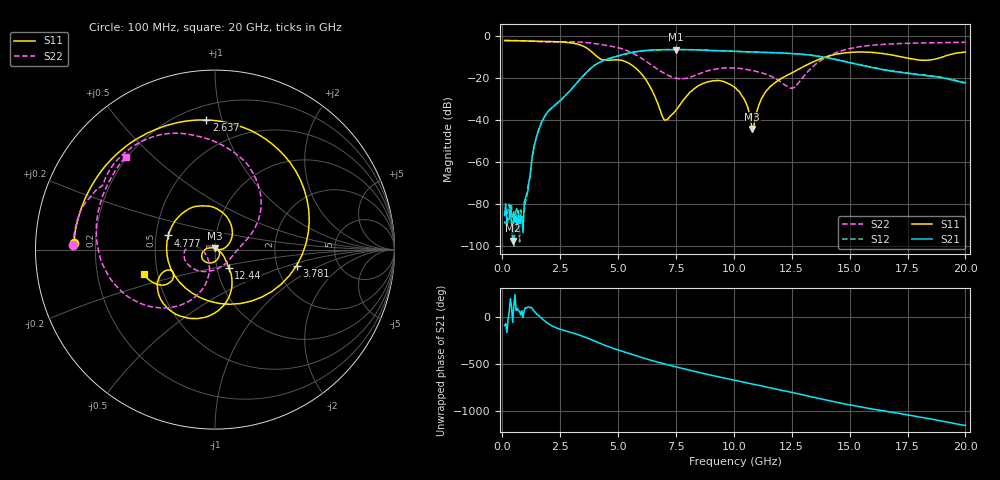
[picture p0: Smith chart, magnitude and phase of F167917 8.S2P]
!  2-Port S-parameters saved by WinCal
! VAR MeasName=S-Parameters (CALIBRATED_DATA) read from VNA (N5242A)
! VAR MeasDate=2016-11-22 9:00:03
! VAR NAME=F167917 8
! VAR FILENAME=F167917 8.S2P
! VAR DATE=2016-11-22 9:00:03
! VAR PHYS_PORTS=1,2
# Hz S DB R 50
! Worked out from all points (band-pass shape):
!   401 points, 100 MHz to 20 GHz, reference 50 ohm
!   highest |S21| = -6.37 dB at 7.513 GHz (marker M1); lowest = -97.2 dB at 448.2 MHz (marker M2)
!   |S21| within 3 dB of the highest: 5.017 GHz to 13.54 GHz (8.526 GHz wide, 91.9 % of centre)
!   lowest |S11| = -44.2 dB at 10.8 GHz (marker M3), VSWR 1.01, Z = 50.1 + j0.616 ohm
!   |S11| at or under -10 dB: 4.127 GHz to 13.93 GHz (9.808 GHz wide, 109 % of centre); 17.32 GHz to 18.97 GHz (1.658 GHz wide, 9.14 % of centre)
!   |S22| runs from -24.7 to -2.0 dB; largest |S21 - S12| = 0.0043
!   S11 on the Smith chart (normalised r, x): 100 MHz: 0.12, +0.02; 2.637 GHz: 0.29, +0.89; 3.781 GHz: 2.57, -0.59; 4.777 GHz: 0.58, +0.10; 12.44 GHz: 1.14, -0.24; 20 GHz: 0.42, -0.14
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1e8  -2.09 177.3  -85.30 -87.7  -87.89 150.7  -2.03 178.3
4.4825e8  -2.13 168.0  -97.22 -53.9  -89.70 -97.5  -2.06 172.4
9.4575e8  -2.21 154.7  -79.15 73.5  -84.02 95.0  -2.18 163.9
1.5925e9  -2.34 135.6  -43.93 12.3  -43.92 11.8  -2.61 153.5
2.63725e9  -2.81 93.9  -29.20 -138.4  -29.20 -138.8  -2.63 138.2
3.43325e9  -4.45 33.9  -19.58 160.7  -19.60 160.6  -2.85 120.0
3.7815e9  -6.69 -11.2  -15.67 127.1  -15.66 127.2  -3.19 110.7
4.1795e9  -10.43 -85.5  -12.59 85.2  -12.53 85.2  -3.81 99.9
4.7765e9  -11.30 163.1  -10.09 29.3  -10.06 28.9  -4.93 82.2
5.92075e9  -16.82 48.1  -7.14 -62.0  -7.16 -62.1  -9.86 38.7
6.7665e9  -33.61 -2.0  -6.45 -123.2  -6.46 -123.3  -16.15 11.0
7.065e9  -39.88 26.2  -6.39 -142.9  -6.41 -142.9  -18.04 -0.6
7.51275e9  -35.02 1.7  -6.37 -171.2  -6.38 -171.3  -20.00 -28.4
8.7565e9  -22.10 -108.4  -6.66 115.2  -6.65 115.2  -16.85 -122.4
1.005e10  -24.40 -176.6  -7.21 45.9  -7.21 46.0  -15.16 -170.8
1.079625e10  -44.18 84.7  -7.53 7.0  -7.51 7.2  -16.30 175.3
1.139325e10  -26.11 -32.2  -7.73 -23.9  -7.72 -23.7  -18.12 170.0
1.2438e10  -17.82 -53.7  -8.21 -79.2  -8.20 -79.2  -24.64 -155.3
1.338325e10  -12.42 -67.5  -9.10 -132.1  -9.08 -131.6  -14.76 -104.6
1.4826e10  -7.90 -107.5  -12.17 151.6  -12.04 152.0  -6.37 -138.6
1.67165e10  -8.72 -150.6  -16.36 69.4  -16.33 69.2  -3.72 179.6
2e10  -7.53 -161.4  -22.25 -76.7  -22.11 -77.3  -2.89 133.6
